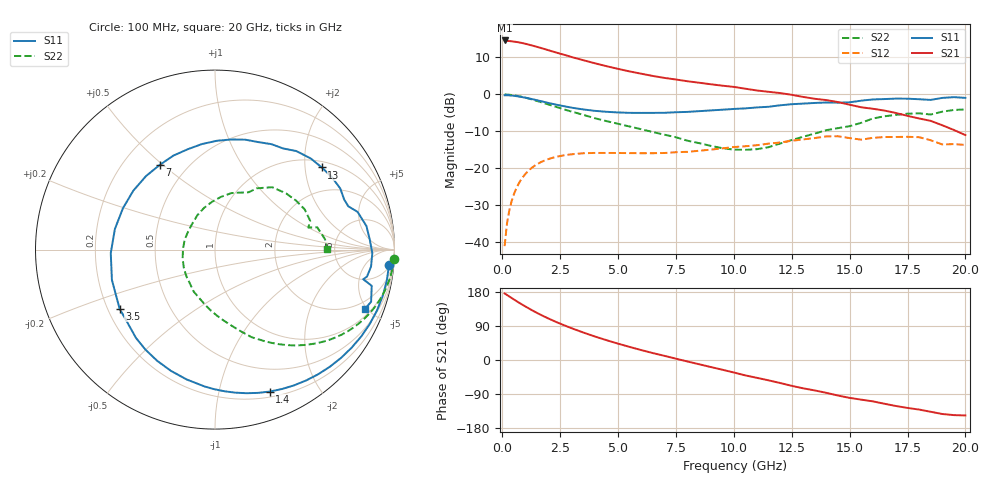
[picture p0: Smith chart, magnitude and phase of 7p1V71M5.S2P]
! Infineon Technologies  Discrete & RF Semiconductors
! bfp620
! VCE =  1.7 V,  IC =  1.5 mA
! Common Emitter S-Parameters:  Sep 2002
# GHz  S  MA  R  50
!  f  S11  S21  S12  S22
! GHz  MAG  ANG  MAG  ANG  MAG  ANG  MAG  ANG
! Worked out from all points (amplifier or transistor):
!   59 points, 100 MHz to 20 GHz, reference 50 ohm
!   highest |S21| = 14.6 dB at 100 MHz (marker M1)
!   |S21| within 3 dB of that: start of sweep to 2.183 GHz
!   unconditionally stable (mu >= 1): 6.054 GHz to 15.71 GHz; 17.68 GHz to end of sweep
!   at 1 GHz: K = 0.13, MSG = 17.6 dB, |S12| = -21.5 dB
!   at 5.5 GHz: K = 0.91, MSG = 11.1 dB, |S12| = -15.9 dB
!   at 20 GHz: K = 1.39, MAG = -2.4 dB, |S12| = -13.7 dB
!   S11 on the Smith chart (normalised r, x): 100 MHz: 6, -21; 1.4 GHz: 0.25, -1.43; 3.5 GHz: 0.25, -0.27; 7 GHz: 0.35, +0.49; 13 GHz: 1.17, +2.45; 20 GHz: 1.41, -4.82
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0.1  0.9734 -5.1  5.375 175.6  0.0088 82.5  0.9988 -2.9
0.3  0.9695 -15.6  5.279 167.7  0.0266 81.3  0.989 -8.7
0.6  0.9474 -30.8  5.135 155.9  0.0529 72.2  0.9602 -16.9
0.8  0.9258 -40.7  5.003 148.4  0.0691 65.9  0.9334 -22.1
1.1  0.8886 -55.1  4.758 137.7  0.0905 56.8  0.8855 -29.4
1.4  0.8476 -68.9  4.49 127.5  0.1082 48.6  0.8328 -35.9
1.8  0.7913 -86.1  4.134 115.1  0.1263 39.0  0.7625 -43.4
2.4  0.7187 -110.0  3.632 98.4  0.1443 27.1  0.6664 -53.0
3  0.6607 -131.7  3.201 83.7  0.1546 17.3  0.5842 -61.2
3.5  0.625 -148.3  2.903 72.5  0.1597 10.4  0.5282 -67.4
4  0.5987 -163.6  2.637 62.0  0.1611 4.3  0.4752 -72.7
5  0.5694 168.3  2.216 43.1  0.1609 -4.1  0.3996 -82.8
6  0.5612 144.1  1.906 26.2  0.1598 -10.0  0.3374 -94.5
7  0.5634 123.1  1.672 11.0  0.1608 -13.6  0.2848 -107.7
8.5  0.5927 97.0  1.439 -11.2  0.1724 -18.4  0.2186 -136.6
10.5  0.6463 67.8  1.193 -40.7  0.1984 -28.7  0.1775 162.2
12  0.7117 50.5  1.042 -60.7  0.2233 -36.6  0.216 116.8
13  0.7506 37.6  0.923 -74.8  0.2456 -44.6  0.2672 93.4
13.5  0.7658 31.9  0.872 -80.4  0.2563 -49.2  0.2951 83.7
15  0.7808 18.0  0.725 -100.0  0.2559 -69.0  0.3709 59.5
17  0.8768 -1.3  0.56 -121.4  0.2649 -82.6  0.5278 31.1
20  0.8976 -21.7  0.281 -146.4  0.2069 -107.3  0.6257 0.4
